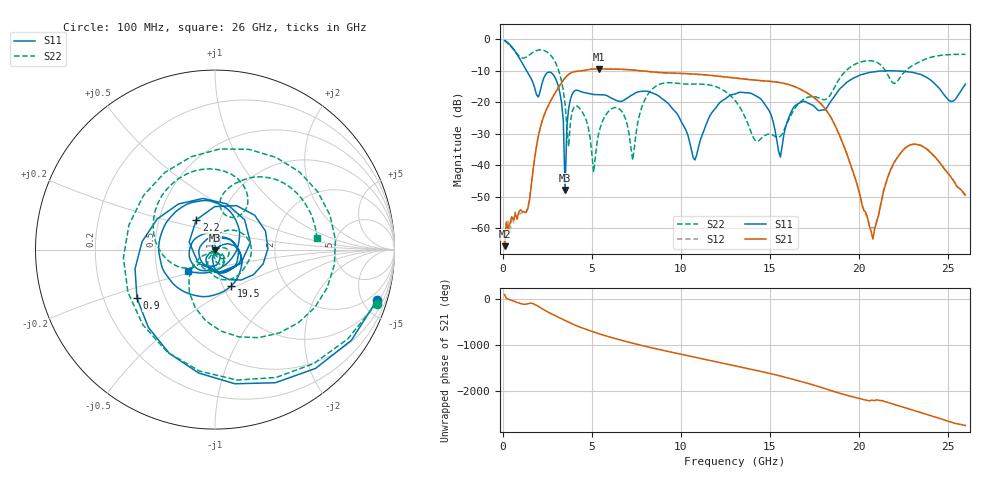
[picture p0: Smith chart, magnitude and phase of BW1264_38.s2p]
!Keysight Technologies,N5245B,MY57181159,A.13.60.06
!Date: Friday, December 18, 2020 23:54:03
!Correction: S11(Full 2 Port(1,2))
!S21(Full 2 Port(1,2))
!S12(Full 2 Port(1,2))
!S22(Full 2 Port(1,2))
!S2P File: Measurements: S11, S21, S12, S22:
# Hz S  dB  R 50
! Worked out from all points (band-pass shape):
!   260 points, 100 MHz to 26 GHz, reference 50 ohm
!   highest |S21| = -9.48 dB at 5.4 GHz (marker M1); lowest = -65.7 dB at 100 MHz (marker M2)
!   |S21| within 3 dB of the highest: 3.48 GHz to 13.19 GHz (9.714 GHz wide, 117 % of centre)
!   lowest |S11| = -47.9 dB at 3.5 GHz (marker M3), VSWR 1.01, Z = 50 - j0.402 ohm
!   |S11| at or under -10 dB: 1.328 GHz to end of sweep
!   |S22| runs from -42.3 to -0.5 dB; largest |S21 - S12| = 0.00056
!   S11 on the Smith chart (normalised r, x): 100 MHz: 1.21, -6.37; 900 MHz: 0.35, -0.25; 2.2 GHz: 0.77, +0.27; 19.5 GHz: 1.10, -0.47; 26 GHz: 0.72, -0.18
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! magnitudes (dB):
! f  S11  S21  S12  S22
! 100 MHz  -0.5  -65.7  -65.1  -0.5
! 900 MHz  -5.8  -54.8  -55.3  -5.3
! 2.2 GHz  -14.2  -26.2  -26.2  -3.5
! 3.2 GHz  -16.9  -14.7  -14.7  -11.1
! 3.4 GHz  -25.9  -13.1  -13.1  -16.4
! 3.5 GHz  -47.9  -12.3  -12.3  -20.7
! 3.7 GHz  -22.0  -11.2  -11.2  -34.1
! 4.5 GHz  -16.9  -10.0  -10.0  -23.5
! 5.1 GHz  -17.6  -9.5  -9.5  -42.3
! 5.4 GHz  -17.7  -9.5  -9.5  -29.6
! 6.6 GHz  -19.8  -9.6  -9.6  -22.4
! 7.3 GHz  -17.7  -9.8  -9.8  -38.4
! 8.8 GHz  -18.2  -10.6  -10.6  -14.4
! 10.8 GHz  -38.4  -11.1  -11.1  -14.3
! 13.1 GHz  -17.4  -12.4  -12.4  -19.8
! 15.6 GHz  -37.5  -13.8  -13.8  -30.9
! 17.4 GHz  -20.9  -18.2  -18.2  -18.3
! 19.5 GHz  -13.1  -39.1  -39.2  -9.0
! 20.8 GHz  -10.4  -63.5  -59.7  -7.0
! 21.7 GHz  -10.1  -42.9  -42.8  -12.0
! 23.3 GHz  -11.0  -33.5  -33.4  -7.6
! 26 GHz  -14.3  -49.5  -49.8  -4.9
